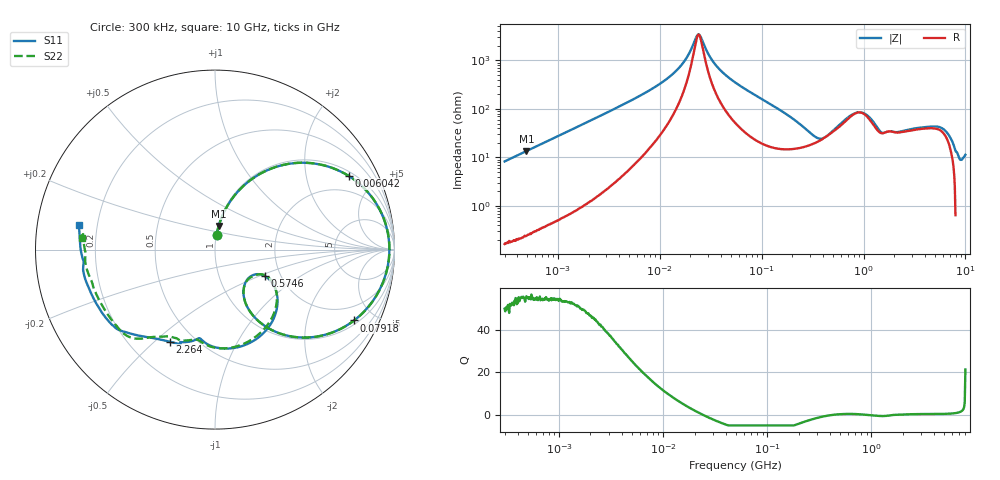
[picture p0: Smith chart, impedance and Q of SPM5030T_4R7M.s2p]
! S-Parameter Data Generated by TDK Corporation
! Copyright(C) 2019 TDK Corporation.
! All Rights Reserved.
! TDK P/N: SPM5030T-4R7M (Inductor)
! Property: L=4.7uH at 100kHz
! Size(LxWxT): 5.2x5x3mm
! Model Type: s2p (Touchstone File Format Version 1.0)
! Frequency: DC=Yes Start=0.3MHz Stop=10000MHz 802points Log-sweep
! Model Generated on Sep. 23, 2019
! Port Assignments:
!  1 ---@@@--- 2
! Applicable Conditions:
!  Temperature = 25 degC
!  DC Bias Current = 0 A
!  Small Signal Operation
! Terms and conditions regarding TDK Simulation Models
! (1)This simulation model is being provided solely for informational purposes. Please refer to the specifications of the products in terms of detailed characteristics of such products.
! (2)In no event shall TDK Corporation of any of its subsidiaries be liable for any loss or damage arising, directly or indirectly,
!  From any information contained in this simulation model, including, but not limited to loss or damages arising from any inaccuracies, omissions or errors in connection with such information.
! (3)Any and all copyrights on this simulation model are owned by TDK Corporation.
!  Duplication or redistribution of this simulation model without prior written permission from TDK Corporation is prohibited.
! (4)This simulation model is subject to any modification or change without any prior notice.
! (5)Neither TDK Corporation nor any of its subsidiaries shall make any warranty, express or implied,
!  Including but not limited to the correctness, implied warranties of merchantability and fitness for a particular purpose with respect to this simulation models.
! (6)The use of this simulation model shall be deemed to have consented to the terms and conditions hereof.
# Hz S MA R 50
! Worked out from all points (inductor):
!   801 points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, 300 kHz to 10 GHz, reference 50 ohm
!   read as one part in series: L = 4.38 uH near 318.3 kHz
!   highest Q = 55.5 at 491.6 kHz (marker M1), where L = 4.38 uH
!   self-resonance near 24.09 MHz
!   S11 on the Smith chart (normalised r, x): 300 kHz: 1.00, +0.16; 6.042 MHz: 1.19, +3.52; 79.18 MHz: 1.18, -3.82; 574.6 MHz: 1.65, -0.54; 2.264 GHz: 0.37, -0.56; 10 GHz: 0.13, +0.09
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300000  0.08194 84.1  0.995 -4.8  0.995 -4.7  0.08194 84.1
491566  0.1334 81.3  0.9886 -7.7  0.9887 -7.7  0.1334 81.2
1713600  0.4222 63.8  0.8979 -25.0  0.898 -25.0  0.4223 63.8
3330145  0.6689 46.3  0.7246 -42.1  0.7246 -42.1  0.669 46.3
6041662  0.8508 28.8  0.4867 -58.5  0.4866 -58.5  0.851 28.8
9671944  0.93 16.8  0.2982 -68.4  0.2983 -68.4  0.9303 16.9
1.626666e7  0.9663 6.1  0.1219 -71.4  0.1219 -71.4  0.9668 6.1
2.41e7  0.9712 -1.1  0.02845 -0.9  0.02847 -0.9  0.9719 -1.1
3.467969e7  0.962 -7.9  0.1135 66.0  0.1135 66.0  0.9629 -7.8
5.477226e7  0.9271 -17.5  0.2613 64.1  0.2613 64.1  0.9283 -17.4
7.918232e7  0.8694 -27.0  0.3997 56.2  0.3997 56.2  0.8709 -26.9
1.563148e8  0.6483 -48.4  0.6674 32.9  0.6674 32.9  0.6502 -48.3
3.126428e8  0.3261 -59.6  0.8038 2.6  0.8038 2.6  0.3282 -59.8
4.329008e8  0.245 -42.0  0.7713 -12.4  0.7714 -12.3  0.2479 -43.5
5.745924e8  0.3129 -28.0  0.683 -23.9  0.683 -23.9  0.2833 -29.0
8.987251e8  0.5123 -51.6  0.4937 -29.1  0.4937 -29.1  0.4906 -49.0
1.24442e9  0.5552 -83.6  0.5403 -25.3  0.5404 -25.3  0.5534 -79.5
1.767019e9  0.5216 -103.4  0.5703 -48.3  0.5703 -48.3  0.5191 -104.2
2.264206e9  0.5719 -116.3  0.5164 -63.4  0.5166 -63.4  0.5487 -118.3
5.930102e9  0.7137 -145.6  0.2348 -114.1  0.2349 -114.1  0.6973 -146.4
8.770142e9  0.7483 -179.8  0.1573 -146.8  0.1572 -146.8  0.734 176.8
1e10  0.7678 169.7  0.1282 -153.7  0.1282 -153.8  0.7463 174.8
